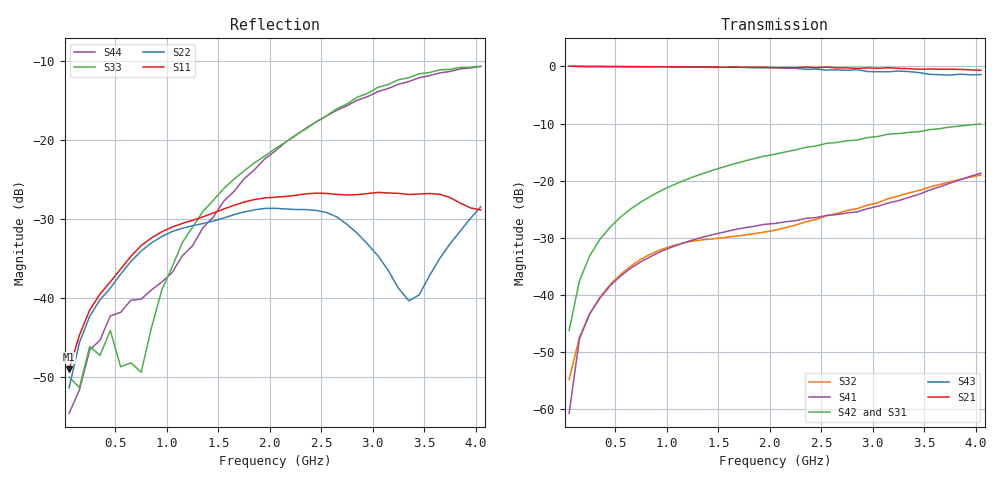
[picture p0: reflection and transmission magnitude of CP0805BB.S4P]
! Network Analyzer HP8720D.07.14 Serial No. US38111185
! 28 Apr 1999  02:06:29
! Frequency 	S11		S21		S31		S41		S12		S22		S23		S24		S13		S23		S33		S34		S14		S24		S34		S44
# HZ  S  DB R 50
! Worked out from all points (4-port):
!   41 points, 50 MHz to 4.05 GHz, reference 50 ohm
!   strongest paths, dB at 50 MHz, 1.05 GHz, 2.05 GHz, 3.05 GHz, 4.05 GHz:
!     S21: 0.0, -0.1, -0.2, -0.3, -0.7
!     S43: 0.0, -0.1, -0.2, -0.9, -1.4
!     S42: -46.3, -20.9, -15.4, -12.3, -10.1
!     S31: -46.8, -20.9, -15.5, -12.4, -10.1
!     S41: -60.8, -31.6, -27.5, -24.5, -18.7
!     S32: -54.9, -31.4, -28.7, -23.9, -19.0
!   lowest |S11| = -49.0 dB at 50 MHz (marker M1), VSWR 1.01, Z = 50.3 - j0.0866 ohm
!   |S11| at or under -10 dB: start of sweep to end of sweep
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5e7  -49.03 -14.1  0.01 -0.5  -49.16 95.9  -57.88 101.5
     0.05 -0.6  -51.34 -15.4  -58.25 36.4  -47.50 94.9
     -46.84 90.6  -54.85 84.7  -49.99 -12.6  0.01 -0.8
     -60.76 79.5  -46.26 76.1  0.03 -0.8  -54.58 -13.7
2.5e8  -41.52 -70.0  -0.01 -3.6  -33.22 85.7  -43.43 86.0
       -0.01 -3.7  -42.32 -65.8  -43.45 86.5  -33.21 85.5
       -33.16 85.8  -43.33 85.2  -46.14 -61.4  -0.00 -4.9
       -43.34 84.6  -33.17 85.8  -0.01 -5.0  -46.58 -42.0
7.5e8  -33.38 -126.5  -0.03 -10.8  -23.75 76.9  -34.17 75.2
       -0.04 -10.8  -34.07 -113.8  -33.77 73.5  -23.72 76.9
       -23.76 76.9  -33.73 73.6  -49.38 146.0  -0.04 -14.6
       -34.19 75.2  -23.72 76.9  -0.05 -14.7  -40.15 -43.7
1.65e9  -28.29 170.6  -0.12 -23.8  -17.16 62.5  -28.60 61.7
        -0.13 -23.5  -29.49 -144.6  -29.71 58.4  -17.04 62.1
        -17.18 62.7  -29.77 58.5  -25.00 60.5  -0.21 -32.3
        -28.60 62.1  -17.07 62.5  -0.15 -32.2  -26.57 -3.5
2.65e9  -26.91 105.4  -0.29 -38.2  -13.36 46.6  -25.92 59.5
        -0.24 -37.8  -29.76 -167.2  -25.68 66.1  -13.21 45.4
        -13.41 47.8  -25.77 67.3  -16.11 -8.7  -0.66 -51.7
        -25.95 60.9  -13.32 46.7  -0.59 -51.5  -16.29 -22.2
3.35e9  -26.93 40.9  -0.31 -48.7  -11.51 38.2  -22.75 66.3
        -0.38 -48.4  -40.37 -126.8  -21.94 64.6  -11.35 36.1
        -11.70 38.3  -22.16 64.7  -12.17 -42.1  -0.89 -63.1
        -22.93 66.3  -11.55 36.0  -0.91 -64.0  -12.66 -47.2
4.05e9  -28.89 -28.4  -0.66 -59.1  -9.79 26.8  -18.42 57.2
        -0.69 -59.0  -28.47 -68.4  -18.79 50.1  -9.77 23.8
        -10.11 29.7  -19.04 53.7  -10.71 -71.3  -1.24 -76.2
        -18.71 59.9  -10.07 26.7  -1.42 -77.1  -10.74 -76.4
